(* Logix 5000 AddOnInstructionDefinition export AMCI_SMD17E2_Preset_Encoder_Position; software revision 20.03 *)

ADD_ON_INSTRUCTION AMCI_SMD17E2_Preset_Encoder_Position   (* revision 1.0, vendor AMCI *)
VAR_INPUT
   save_in_flash_0_no_1_yes : BOOL; {required}
   Target_Position : DINT; {required}
END_VAR
VAR_IN_OUT
   AMCI_SMD17E2_output_data : _000A:SMD17E2_788832CB:O:0; {required}
END_VAR
VAR
   Upper_Result_X_1000 : DINT;
   command_data_block : INT[10];
        [0]   // Command Bits MSW
        [1]   // Command Bits LSW
        [2]   // Upper Target Position
        [3]   // Lower Target Position
        [4]   // Upper Programmed Speed
        [5]   // Lower Programmed Speed
END_VAR

ROUTINE Logic   (* ladder *)
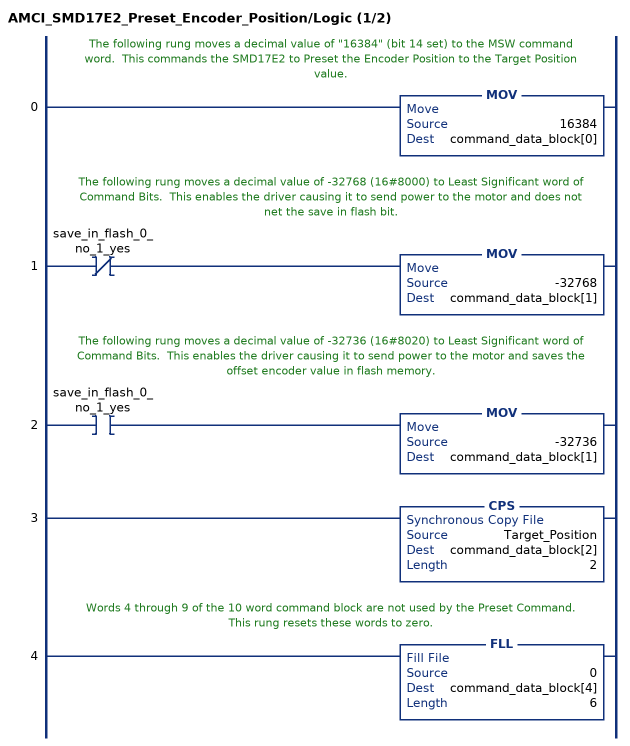
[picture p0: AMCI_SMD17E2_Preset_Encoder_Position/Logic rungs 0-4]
   // The following rung moves a decimal value of "16384" (bit 14 set) to the MSW command word.  This commands the SMD17E2 to Preset the Encoder Position to the Target Position value.
   0: MOV(16384,command_data_block[0]);
   // The following rung moves a decimal value of -32768 (16#8000) to Least Significant word of Command Bits.  This enables the driver causing it to send power to the motor and does not net the save in flash bit.
   1: XIO(save_in_flash_0_no_1_yes)MOV(-32768,command_data_block[1]);
   // The following rung moves a decimal value of -32736 (16#8020) to Least Significant word of Command Bits.  This enables the driver causing it to send power to the motor and saves the offset encoder value in flash memory.
   2: XIC(save_in_flash_0_no_1_yes)MOV(-32736,command_data_block[1]);
   3: CPS(Target_Position,command_data_block[2],2);
   // Words 4 through 9 of the 10 word command block are not used by the Preset Command.  This rung resets these words to zero.
   4: FLL(0,command_data_block[4],6);
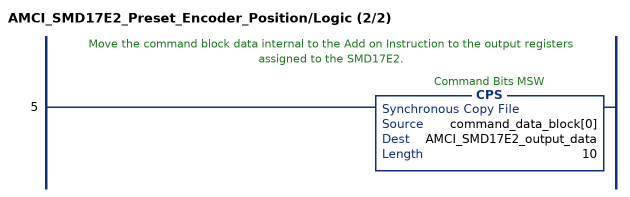
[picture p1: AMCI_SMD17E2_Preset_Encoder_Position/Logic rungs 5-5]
   // Move the command block data internal to the Add on Instruction to the output registers assigned to the SMD17E2.
   5: CPS(command_data_block[0],AMCI_SMD17E2_output_data,10);
END_ROUTINE
END_ADD_ON_INSTRUCTION
